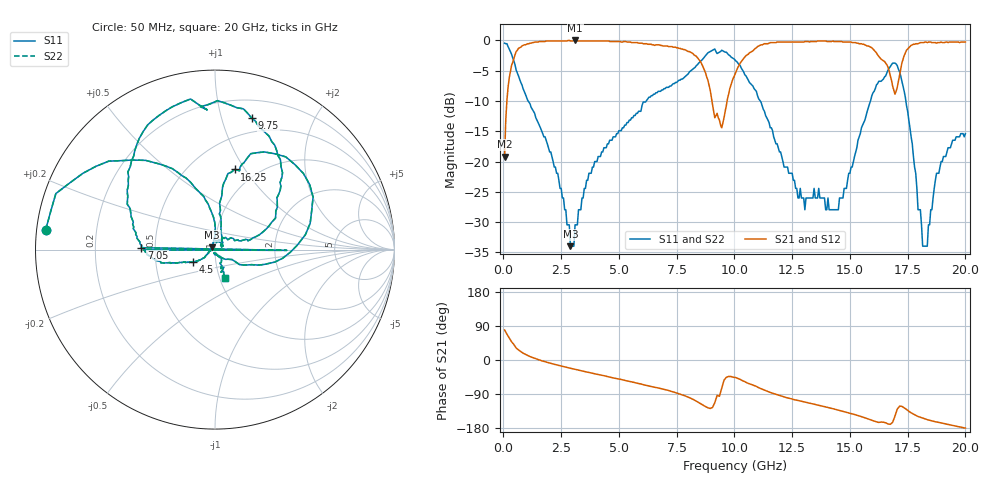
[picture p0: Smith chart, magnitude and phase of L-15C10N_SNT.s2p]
#	mhz	s	ma	r	50
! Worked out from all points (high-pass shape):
!   400 points, 50 MHz to 20 GHz, reference 50 ohm
!   highest |S21| = 0.00 dB at 3.1 GHz (marker M1); lowest = -19.2 dB at 50 MHz (marker M2)
!   |S21| within 3 dB of the highest: 448 MHz to 8.43 GHz (7.982 GHz wide, 180 % of centre); 10.39 GHz to 16.33 GHz (5.935 GHz wide, 44.4 % of centre)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
!   lowest |S11| = -34.0 dB at 2.9 GHz (marker M3), VSWR 1.04, Z = 48.5 + j1.28 ohm
!   |S11| at or under -10 dB: 1.069 GHz to 6.181 GHz (5.113 GHz wide, 141 % of centre); 11.12 GHz to 15.89 GHz (4.772 GHz wide, 35.3 % of centre); 17.42 GHz to end of sweep
!   |S22| runs from -34.0 to -0.4 dB; largest |S21 - S12| = 0
!   S11 on the Smith chart (normalised r, x): 50 MHz: 0.03, +0.06; 4.5 GHz: 0.78, -0.11; 7.05 GHz: 0.42, +0.01; 9.75 GHz: 0.36, +1.25; 16.25 GHz: 0.79, +0.90; 20 GHz: 1.06, -0.35
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50  0.95 173.4  0.11 79.3  0.11 79.3  0.95 173.4
550  0.57 123.1  0.81 31.6  0.81 31.6  0.57 123.1
2900  0.02 138.9  0.99 -21.8  0.99 -21.8  0.02 138.9
3100  0.03 2.2  1 -24.6  1 -24.6  0.03 2.2
3400  0.05 -150.0  0.99 -28.8  0.99 -28.8  0.05 -150.0
4500  0.14 -150.3  0.99 -43.8  0.99 -43.8  0.14 -150.3
6700  0.38 -175.7  0.92 -73.8  0.92 -73.8  0.38 -175.7
6950  0.4 -179.8  0.9 -77.3  0.9 -77.3  0.4 -179.8
7000  0.4 -0.6  0.9 -78.1  0.9 -78.1  0.4 -0.6
7050  0.41 178.5  0.9 -79.0  0.9 -79.0  0.41 178.5
8750  0.75 124.2  0.54 -123.0  0.54 -123.0  0.75 124.2
9450  0.83 89.0  0.19 -74.0  0.19 -74.0  0.83 89.0
9750  0.76 74.3  0.36 -43.4  0.36 -43.4  0.76 74.3
10050  0.68 62.3  0.54 -46.3  0.54 -46.3  0.68 62.3
11300  0.26 18.4  0.94 -79.5  0.94 -79.5  0.26 18.4
13350  0.05 81.9  0.98 -115.1  0.98 -115.1  0.05 81.9
14500  0.04 24.2  0.98 -132.2  0.98 -132.2  0.04 24.2
16250  0.46 76.2  0.74 -164.8  0.74 -164.8  0.46 76.2
16700  0.59 66.3  0.56 -169.3  0.56 -169.3  0.59 66.3
17400  0.34 -11.8  0.79 -128.3  0.79 -128.3  0.34 -11.8
18150  0.02 -79.0  0.96 -153.2  0.96 -153.2  0.02 -79.0
20000  0.17 -70.3  0.97 -179.5  0.97 -179.5  0.17 -70.3
